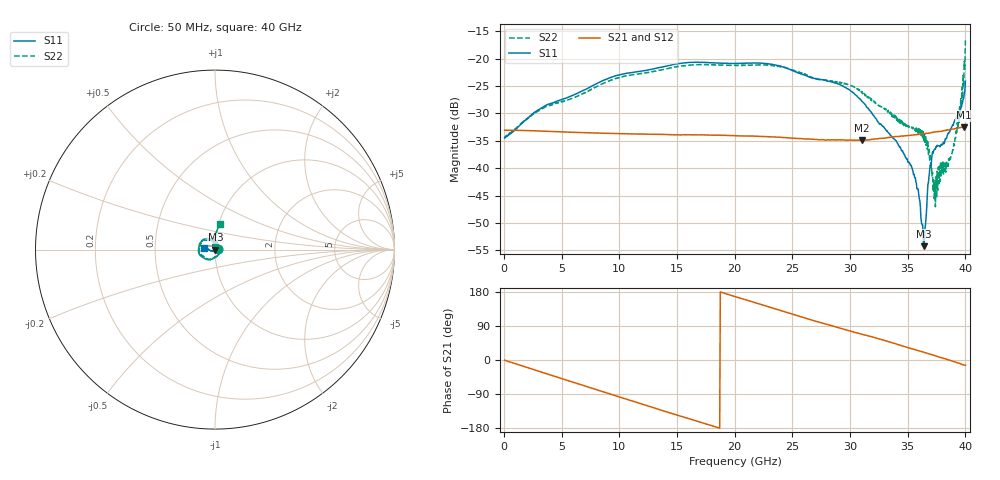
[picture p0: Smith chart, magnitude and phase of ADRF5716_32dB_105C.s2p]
! Device: ADRF5716
! Description: 30GHz 2-Bit Digital Attenuator
! Frequency: 100 MHz – 30 GHz
! Ports:
! ATTIN  = Port 1
! ATTOUT = Port 2
! State: 32 dB Attenuation selected
! Supply Voltage:
! VDD  =  +3.30 Volts
! VSS  =  -3.30 Volts
! Control Voltages:
! D5 = 0V, D6 = 3.3V
! Temperature = +105 C
! Data: Data was collected using a calibrated network analyzer.
!  The reference plane is the package pins of ADRF5716 switch.
! Note: Analog Devices supplies this data as a sample of measured data for this product.
!  Your particular data for this product may vary.
!  Analog Devices reserves the right to change this data at anytime
# HZ S DB R 50
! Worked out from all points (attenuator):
!   800 points, 50 MHz to 40 GHz, reference 50 ohm
!   highest |S21| = -32.51 dB at 39.85 GHz (marker M1); lowest = -34.9 dB at 31 GHz (marker M2)
!   lowest |S11| = -54.2 dB at 36.4 GHz (marker M3), VSWR 1.00, Z = 50.2 - j0.0355 ohm
!   |S11| at or under -10 dB: start of sweep to end of sweep
!   |S22| runs from -47.0 to -16.7 dB; largest |S21 - S12| = 0
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5e7  -34.47 4.2  -33.05 -0.5  -33.05 -0.5  -34.49 4.4
2.8e9  -29.56 -52.1  -33.18 -27.8  -33.18 -27.8  -29.67 -49.6
6.75e9  -25.91 -101.0  -33.49 -66.0  -33.49 -66.0  -26.49 -100.5
1.34e10  -21.63 -150.7  -33.79 -130.2  -33.79 -130.2  -22.13 -153.2
2.005e10  -20.87 169.5  -34.06 167.1  -34.06 167.1  -21.19 164.3
2.67e10  -23.50 130.5  -34.69 105.2  -34.69 105.2  -23.48 119.1
2.915e10  -24.76 115.2  -34.79 83.9  -34.79 83.9  -24.43 104.4
3.1e10  -27.69 98.0  -34.90 68.3  -34.90 68.3  -26.22 84.0
3.335e10  -33.61 93.7  -34.37 48.6  -34.37 48.6  -29.82 66.5
3.545e10  -40.51 85.3  -33.96 28.8  -33.96 28.8  -32.52 48.9
3.585e10  -43.72 82.8  -33.86 25.3  -33.86 25.3  -32.68 42.9
3.625e10  -50.34 49.3  -33.74 21.9  -33.74 21.9  -33.18 36.0
3.64e10  -54.22 -10.5  -33.69 20.5  -33.69 20.5  -34.94 31.5
3.655e10  -50.16 -68.0  -33.66 19.1  -33.66 19.1  -34.04 28.1
3.695e10  -39.45 -116.9  -33.56 15.4  -33.56 15.4  -37.69 20.2
3.72e10  -37.25 -135.6  -33.42 12.8  -33.42 12.8  -44.20 5.3
3.74e10  -36.52 -145.8  -33.35 11.2  -33.35 11.2  -47.03 35.1
3.785e10  -35.96 -156.6  -33.27 6.4  -33.27 6.4  -38.77 79.9
3.89e10  -32.07 -167.1  -32.85 -3.2  -32.85 -3.2  -36.65 74.4
3.955e10  -29.38 -179.9  -32.60 -9.7  -32.60 -9.7  -30.37 109.0
3.985e10  -27.27 170.8  -32.51 -13.0  -32.51 -13.0  -25.06 96.4
4e10  -24.13 169.6  -32.56 -14.2  -32.56 -14.2  -16.68 79.7
